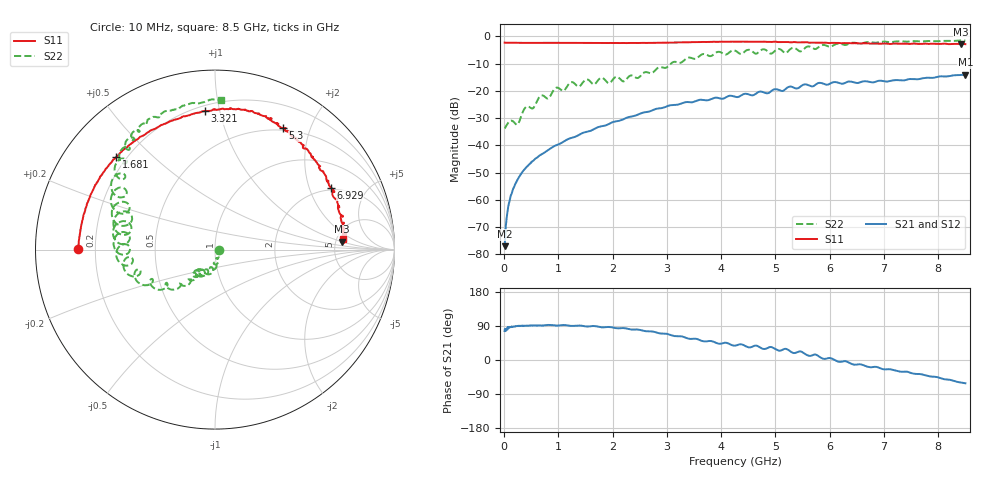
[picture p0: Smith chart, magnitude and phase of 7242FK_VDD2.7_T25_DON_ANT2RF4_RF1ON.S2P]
!Agilent Technologies,E5071C,MY46417908,A.11.23
!Date: Wed Dec 09 15:39:00 2020
!Data & Calibration Information:
!Freq	S11:SOLT2(ON)	S21:SOLT2(ON)	S12:SOLT2(ON)	S22:SOLT2(ON)
!PortZ  Port1:50+j0  Port2:50+j0
!Above PortZ is port z conversion or system Z0 setting when saving the data.
!When reading, reference impedance value at option line is always used.
# Hz S dB R 50
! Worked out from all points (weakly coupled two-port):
!   1601 points, 10 MHz to 8.5 GHz, reference 50 ohm
!   highest |S21| = -14.05 dB at 8.5 GHz (marker M1); lowest = -77.0 dB at 10 MHz (marker M2)
!   lowest |S11| = -3.0 dB at 8.42 GHz (marker M3), VSWR 5.89, Z = 285 + j51.2 ohm
!   |S11| at or under -10 dB: nowhere
!   |S22| runs from -33.8 to -1.5 dB; largest |S21 - S12| = 0.003
!   S11 on the Smith chart (normalised r, x): 10 MHz: 0.13, +0.00; 1.681 GHz: 0.16, +0.39; 3.321 GHz: 0.23, +0.90; 5.3 GHz: 0.48, +1.60; 6.929 GHz: 1.89, +2.81; 8.5 GHz: 5.73, +1.35
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1e7  -2.34 179.7  -76.99 76.4  -79.85 75.2  -33.79 -0.6
6.30625e7  -2.38 178.1  -64.24 80.5  -64.45 84.8  -32.10 -18.1
1.108188e8  -2.38 176.8  -59.49 87.3  -59.59 85.9  -31.09 -38.2
2.43475e8  -2.41 173.1  -52.69 89.6  -52.79 89.5  -32.40 -59.1
3.336812e8  -2.42 170.6  -49.88 90.3  -49.95 90.3  -28.33 -54.2
9.545125e8  -2.43 154.4  -40.05 91.0  -40.03 91.1  -18.93 -94.8
1.426769e9  -2.42 143.3  -35.67 90.5  -35.66 90.5  -17.59 -106.7
1.681469e9  -2.44 136.9  -33.77 89.5  -33.77 89.5  -17.41 -115.5
1.7929e9  -2.45 133.8  -33.00 86.3  -33.00 86.4  -15.24 -121.3
1.930862e9  -2.46 130.3  -32.17 87.2  -32.17 87.2  -17.26 -126.0
2.461488e9  -2.49 116.0  -28.77 80.3  -28.78 80.3  -15.33 -128.9
2.843538e9  -2.41 105.3  -26.45 71.1  -26.46 71.1  -11.48 -130.7
3.3211e9  -2.22 94.3  -24.25 60.2  -24.25 60.2  -8.75 -142.7
4.255e9  -2.00 77.3  -22.17 37.9  -22.18 37.8  -5.26 -179.9
5.172981e9  -2.14 63.9  -19.57 29.5  -19.56 29.3  -6.12 159.1
5.300331e9  -2.22 60.7  -18.52 20.3  -18.49 20.4  -4.38 161.9
5.671769e9  -2.31 54.1  -18.40 12.0  -18.34 11.9  -4.13 146.3
6.92935e9  -2.72 28.2  -16.29 -22.1  -16.33 -21.8  -2.09 126.5
7.088538e9  -2.77 25.8  -16.52 -24.2  -16.57 -24.2  -2.12 122.5
7.773044e9  -2.70 11.8  -15.24 -40.6  -15.26 -40.6  -1.78 111.6
8.420406e9  -2.98 3.6  -14.20 -59.4  -14.28 -59.7  -1.56 90.4
8.5e9  -2.89 4.6  -14.05 -61.4  -14.15 -61.3  -1.57 87.6
